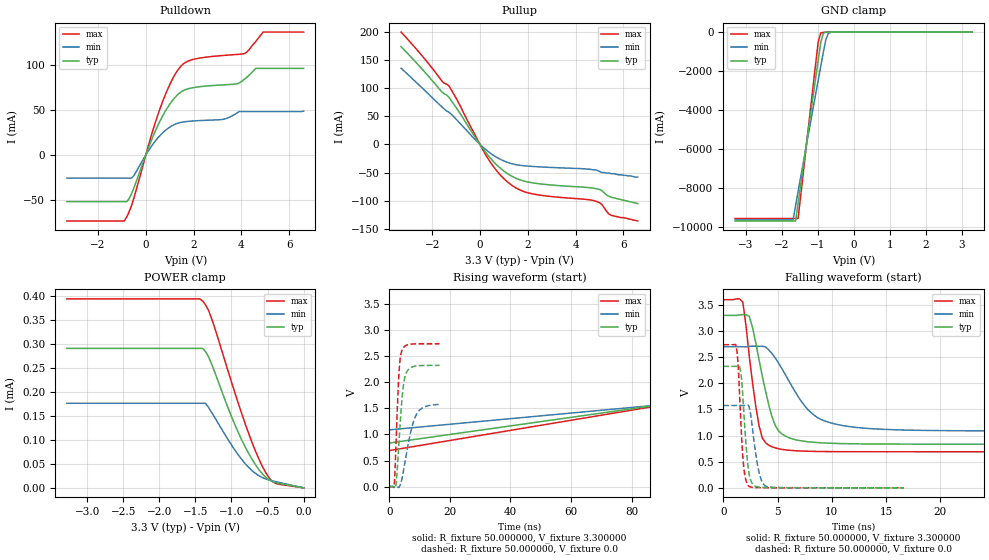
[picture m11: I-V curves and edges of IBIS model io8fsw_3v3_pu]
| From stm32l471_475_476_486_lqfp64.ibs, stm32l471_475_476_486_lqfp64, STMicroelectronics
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|   Model io8fsw_3v3_pu
[Model]  io8fsw_3v3_pu
Model_type I/O
Polarity   Non-Inverting
Enable   Active-Low
Vinl =   0.990000V
Vinh =   2.310000V
Vmeas =  1.650000V
Cref =   100.000000nF
Rref =   1.000000k
Vref =   3.300000V
C_comp   2.968600pF   2.938100pF   3.196200pF
[Temperature Range]   25.000000   0.125000k   -40.000000
[Pullup Reference]   3.300000V   2.700000V   3.600000V
[Pulldown Reference]   0.0V   0.0V   0.0V
[POWER Clamp Reference]   3.300000V   2.700000V   3.600000V
[GND Clamp Reference]   0.0V   0.0V   0.0V
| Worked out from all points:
|   slope of the pulldown table from 0 to 0.495 V, typ, clamps not added: 15.4 ohm
|   slope of the pullup table from 0 to 0.495 V, typ, clamps not added: 18.1 ohm
|   GND clamp passes 1 mA (typ) near -0.58 V on its own axis
|   rising waveform, R_fixture 50.000000, V_fixture 3.300000: 20-80 % time 180ns typ, 180ns min, 180ns max; typ from 0.836 V to 3.3 V
|   rising waveform, R_fixture 50.000000, V_fixture 0.0: 20-80 % time 1.71ns typ, 3.36ns min, 1.18ns max; typ from 0.001 V to 2.33 V
|   falling waveform, R_fixture 50.000000, V_fixture 3.300000: 20-80 % time 1.58ns typ, 3.13ns min, 1.09ns max; typ from 3.3 V to 0.836 V
|   falling waveform, R_fixture 50.000000, V_fixture 0.0: 20-80 % time 488ps typ, 660ps min, 410ps max; typ from 2.33 V to 0.001 V
[Pulldown]
|Voltage   I(typ)   I(min)   I(max)
-3.3V     -51.62mA   -25.53mA   -73.04mA
-900mV    -51.62mA   -25.53mA   -73.04mA
-500mV    -36.51mA   -22.79mA   -47.71mA
200mV     14.02mA    8.316mA    18.9mA
700mV     42.98mA    24.4mA     58.9mA
1.2V      63.06mA    33.8mA     88.14mA
1.6V      71.63mA    36.67mA    101.4mA
3.2V      77.51mA    39.29mA    110mA
4.1V      83.28mA    47.99mA    112mA
4.6V      95.81mA    47.99mA    125.7mA
4.9V      95.81mA    47.99mA    136mA
6.6V      95.81mA    48.43mA    136mA
[Pullup]
|Voltage   I(typ)   I(min)   I(max)
-3.3V     173.5mA    135.3mA    199.5mA
-1.6V     93.59mA    66.94mA    113mA
-1.3V     83.83mA    57.27mA    104.1mA
300mV     -17.49mA   -11.19mA   -22.71mA
700mV     -36.32mA   -22.9mA    -46.84mA
1.2V      -53.2mA    -32.62mA   -68.33mA
1.7V      -63.36mA   -37.26mA   -81.47mA
2.2V      -68.23mA   -39.11mA   -87.81mA
4.8V      -78.1mA    -45mA      -100.2mA
5.1V      -82mA      -50mA      -106.7mA
5.5V      -94mA      -52mA      -126mA
6.6V      -105mA     -58mA      -136mA
[GND_clamp]
|Voltage   I(typ)   I(min)   I(max)
-3.3V     -9.687A    -9.633A    -9.557A
-1.69V    -9.687A    -9.633A    -9.557A
-1.62V    -9.687A    -8.894A    -9.557A
-1.55V    -8.764A    -8.167A    -9.557A
-1.13V    -3.236A    -3.867A    -2.713A
-990mV    -1.416A    -2.448A    -480.1mA
-920mV    -530mA     -1.746A    -39.96mA
-850mV    -62.36mA   -1.055A    -14.04mA
-780mV    -12.04mA   -390.4mA   -9.013mA
-710mV    -4.897mA   -69.08mA   -5.32mA
-640mV    -2.305mA   -14.59mA   -2.498mA
3.28V     0A         0A         0A
[POWER_clamp]
|Voltage   I(typ)   I(min)   I(max)
-3.28V    291uA      176.5uA    394.3uA
-1.44V    291uA      176.5uA    394.3uA
-1.4V     291uA      176.5uA    389.8uA
-1.36V    284.6uA    176.5uA    382.1uA
-1.28V    260.2uA    158.7uA    355.4uA
-1V       148.8uA    89.45uA    220.9uA
-840mV    94.39uA    55.87uA    146.9uA
-680mV    51.08uA    31.49uA    81.3uA
-560mV    27.28uA    20.64uA    41.26uA
-480mV    16.8uA     16.48uA    21.17uA
-400mV    11.23uA    13.43uA    10.02uA
0V        0A         5.022nA    0A
[Ramp]
| variable   typ   min   max
dV/dt_r  1.39450/1.70870n   0.94482/3.37594n   1.64288/1.17422n
dV/dt_f  1.47838/1.57323n   0.96678/3.12576n   1.74562/1.07832n
R_load = 50.000000
[Rising Waveform]
R_fixture= 50.000000
V_fixture= 3.300000
V_fixture_min= 2.700000
V_fixture_max= 3.600000
|time   V(typ)   V(min)   V(max)
0s        836mV      1.089V     690.6mV
300.3ns   3.3V       2.7V       3.6V
600.6ns   3.3V       2.7V       3.6V
29.73us   3.3V       2.7V       3.6V
[Rising Waveform]
R_fixture= 50.000000
V_fixture= 0.0
V_fixture_min= 0.0
V_fixture_max= 0.0
|time   V(typ)   V(min)   V(max)
0s        932.4uV    1.399mV    660.9uV
1.635ns   -2.523mV   1.4mV      2.87mV
2.236ns   36.83mV    1.59mV     796.5mV
3.136ns   766.3mV    -16.86mV   2.077V
3.604ns   1.201V     28.39mV    2.446V
4.104ns   1.598V     125.9mV    2.594V
5.439ns   2.153V     545.7mV    2.704V
7.174ns   2.283V     1.065V     2.732V
8.909ns   2.313V     1.376V     2.737V
16.62ns   2.325V     1.576V     2.739V
[Falling Waveform]
R_fixture= 50.000000
V_fixture= 3.300000
V_fixture_min= 2.700000
V_fixture_max= 3.600000
|time   V(typ)   V(min)   V(max)
0s        3.3V       2.7V       3.6V
1.802ns   3.315V     2.7V       3.552V
2.402ns   3.279V     2.709V     2.502V
3.003ns   2.768V     2.709V     1.546V
3.604ns   2.125V     2.708V     951.8mV
4.805ns   1.187V     2.481V     764.2mV
6.006ns   963.7mV    2.063V     720.8mV
9.009ns   862.3mV    1.309V     695.8mV
15.92ns   837.7mV    1.111V     691mV
149.5ns   836mV      1.089V     690.6mV
[Falling Waveform]
R_fixture= 50.000000
V_fixture= 0.0
V_fixture_min= 0.0
V_fixture_max= 0.0
|time   V(typ)   V(min)   V(max)
0s        2.325V     1.576V     2.739V
1.201ns   2.325V     1.576V     2.696V
1.368ns   2.33V      1.576V     2.34V
1.568ns   2.263V     1.576V     1.468V
1.835ns   1.635V     1.576V     504.2mV
2.102ns   804.7mV    1.581V     136.5mV
2.336ns   325.6mV    1.571V     33.92mV
3.237ns   16.16mV    352.6mV    5.547mV
3.871ns   7.492mV    37.75mV    3.459mV
16.62ns   932.4uV    1.399mV    660.9uV
